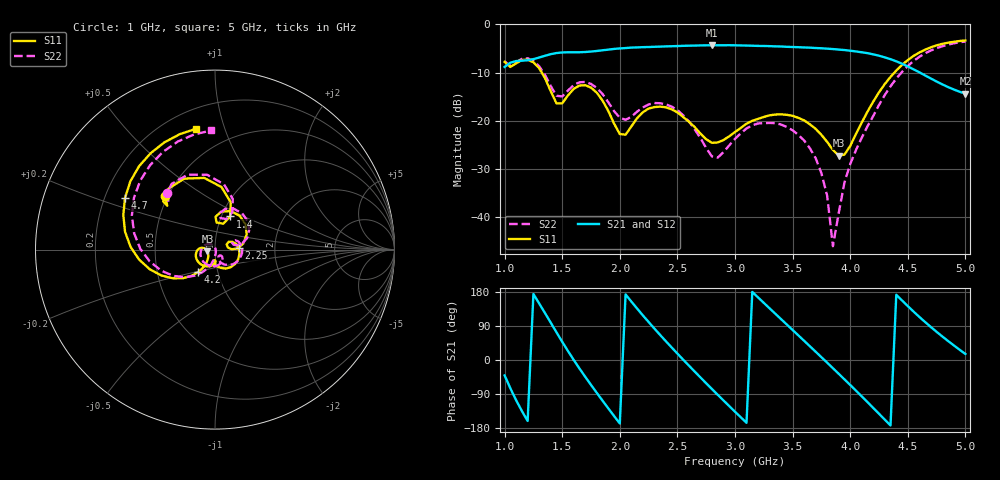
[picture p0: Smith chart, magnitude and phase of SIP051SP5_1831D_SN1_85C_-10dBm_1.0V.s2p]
# GHz  S  dB  R  50
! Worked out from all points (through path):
!   81 points, 1 GHz to 5 GHz, reference 50 ohm
!   highest |S21| = -4.32 dB at 2.8 GHz (marker M1); lowest = -14.4 dB at 5 GHz (marker M2)
!   lowest |S11| = -27.3 dB at 3.9 GHz (marker M3), VSWR 1.09, Z = 45.9 - j0.842 ohm
!   |S11| at or under -10 dB: 1.322 GHz to 4.384 GHz (3.062 GHz wide, 107 % of centre)
!   |S22| runs from -46.1 to -3.6 dB; largest |S21 - S12| = 0.0021
!   S11 on the Smith chart (normalised r, x): 1 GHz: 0.49, +0.35; 1.4 GHz: 1.10, +0.42; 2.25 GHz: 1.31, +0.02; 4.2 GHz: 0.80, -0.21; 4.7 GHz: 0.28, +0.25; 5 GHz: 0.32, +0.80
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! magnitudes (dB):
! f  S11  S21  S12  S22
! 1 GHz  -7.8  -8.8  -8.8  -7.7
! 1.25 GHz  -7.9  -7.2  -7.2  -7.6
! 1.4 GHz  -13.8  -6.2  -6.2  -12.8
! 1.5 GHz  -16.4  -5.8  -5.8  -15.0
! 1.7 GHz  -12.6  -5.7  -5.7  -12.0
! 1.85 GHz  -15.8  -5.4  -5.4  -14.5
! 2 GHz  -22.8  -5.0  -5.0  -19.4
! 2.25 GHz  -17.5  -4.7  -4.7  -16.6
! 2.35 GHz  -17.1  -4.6  -4.6  -16.4
! 2.55 GHz  -19.2  -4.5  -4.4  -18.9
! 2.8 GHz  -24.6  -4.3  -4.3  -27.5
! 3 GHz  -22.4  -4.3  -4.3  -23.8
! 3.35 GHz  -18.7  -4.6  -4.5  -20.5
! 3.7 GHz  -21.7  -4.9  -4.9  -27.8
! 3.8 GHz  -24.4  -5.0  -5.0  -35.6
! 3.85 GHz  -26.1  -5.1  -5.1  -46.1
! 3.9 GHz  -27.3  -5.2  -5.2  -39.3
! 4 GHz  -25.3  -5.5  -5.5  -29.0
! 4.2 GHz  -16.0  -6.2  -6.2  -19.0
! 4.35 GHz  -10.9  -7.2  -7.2  -12.9
! 4.7 GHz  -4.8  -11.2  -11.2  -5.4
! 5 GHz  -3.3  -14.4  -14.4  -3.6
